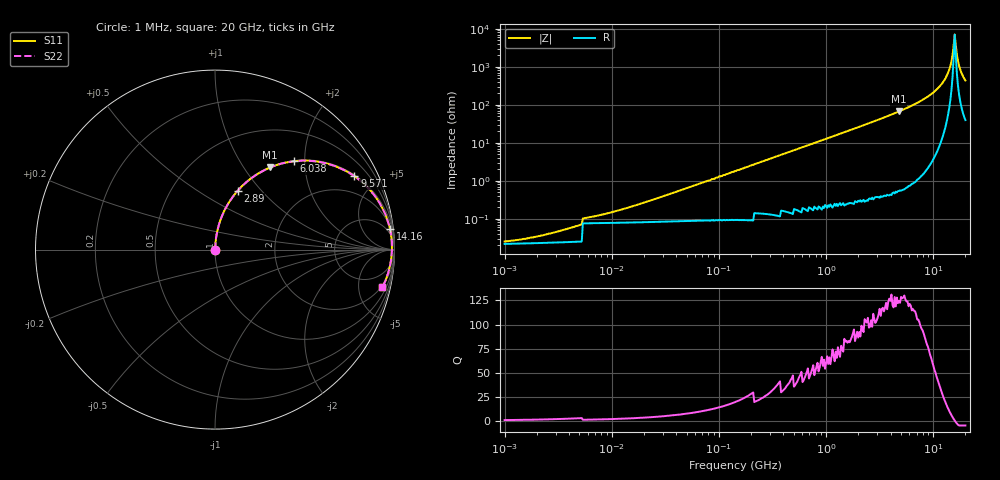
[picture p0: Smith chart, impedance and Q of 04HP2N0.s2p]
# MHz S MA R 50
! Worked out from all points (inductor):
!   431 points, 1 MHz to 20 GHz, reference 50 ohm
!   read as one part in series: L = 2 nH near 19.51 MHz
!   highest Q = 127 at 4.796 GHz (marker M1), where L = 2.2 nH
!   self-resonance near 15.89 GHz
!   S11 on the Smith chart (normalised r, x): 1 MHz: 1.00, +0.00; 2.89 GHz: 1.01, +0.75; 6.038 GHz: 1.01, +1.77; 9.571 GHz: 1.06, +3.77; 14.16 GHz: 3, +17; 20 GHz: 1.77, -8.64
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1  0.0004499 16.2  1 -0.0  1 -0.0  0.0004499 16.2
2.455  0.0005551 33.7  1 -0.0  1 -0.0  0.0005551 33.7
5.25  0.0008272 52.8  1 -0.0  1 -0.0  0.0008272 52.8
27.564  0.003523 79.1  0.999 -0.2  0.999 -0.2  0.003523 79.1
144.716  0.018 85.8  0.999 -1.0  0.999 -1.0  0.018 85.8
742.485  0.093 83.6  0.994 -5.3  0.994 -5.3  0.093 83.6
2889.541  0.35 69.0  0.933 -20.5  0.933 -20.5  0.35 69.0
3898.162  0.461 62.1  0.884 -27.4  0.884 -27.4  0.461 62.1
4796.026  0.551 56.1  0.83 -33.4  0.83 -33.4  0.551 56.1
6038.171  0.661 48.2  0.745 -41.3  0.745 -41.3  0.661 48.2
9570.912  0.878 27.8  0.466 -61.4  0.466 -61.4  0.878 27.8
12330.47  0.959 14.3  0.248 -73.5  0.248 -73.5  0.959 14.3
14157.74  0.982 6.6  0.116 -77.6  0.116 -77.6  0.982 6.6
14825.14  0.985 4.0  0.071 -75.9  0.071 -75.9  0.985 4.0
15170.55  0.986 2.7  0.049 -72.1  0.049 -72.1  0.986 2.7
15524  0.986 1.4  0.028 -60.2  0.028 -60.2  0.986 1.4
15885.69  0.986 0.1  0.014 -8.7  0.014 -8.7  0.986 0.1
16634.54  0.984 -2.5  0.046 68.4  0.046 68.4  0.984 -2.5
17418.69  0.98 -5.1  0.09 74.6  0.09 74.6  0.98 -5.1
17824.53  0.977 -6.3  0.112 75.1  0.112 75.1  0.977 -6.3
19099.64  0.966 -10.2  0.178 73.8  0.178 73.8  0.966 -10.2
20000  0.956 -12.7  0.221 72.1  0.221 72.1  0.956 -12.7
